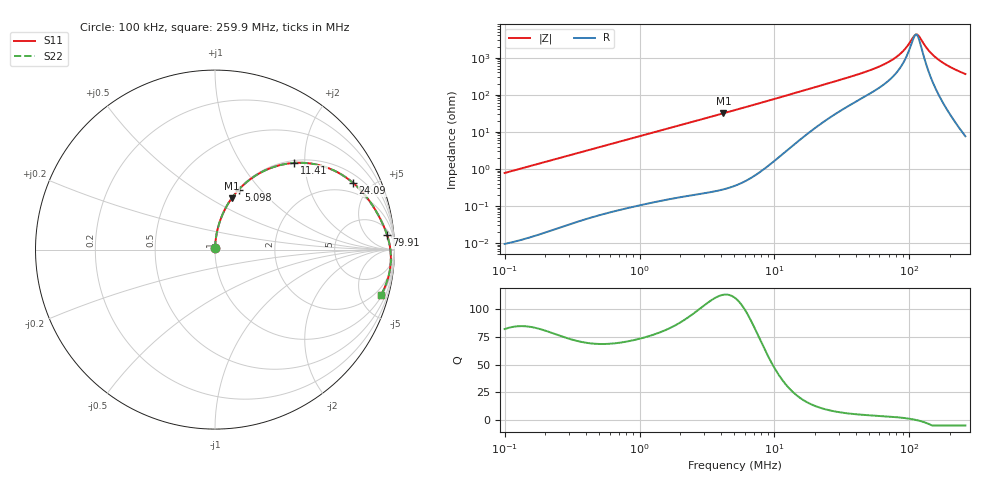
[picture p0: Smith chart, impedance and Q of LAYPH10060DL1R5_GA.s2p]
! LAYPH10060DL1R5_GA  S-PARAMETER MODEL  ( General Type )
! Model Generated by TAIYO YUDEN Corporation (http://www.ty-top.com)
! Version 3.0
! TAIYO YUDEN Control No. 180828NI43SB-FBB
! Copyright(c) 2017 TAIYO YUDEN CO.,LTD. All Rights Reserved.
! Product Description (link to TY-COMPAS)
! https://ds.yuden.co.jp/TYCOMPAS/or/detail?pn=LAYPH10060DL1R5NGA&u=M
! Products Name : Inductors
! Characteristics :
!  Inductance : 1.5 uH , SRF(min) : -Hz , DC Resistance(max) : 0.007 Ohm
!  Rated Current : Saturation :9 A , Temp Rise : 5.6 A (25 degC)
!  Case Size : 10.1 x 10.0 / 0.398 x 0.394 [mm/inch] , Thickness : 6 / 0.236 [mm/inch]
!  (Conditions: Temperature = 25 degC , DC Bias Current/Voltage = 0A / 0V)
! External Node Assignments :
!  1  o---GGG---o  2
! GND o---------o GND
! Frequency Range : 0.1MHz  -  259.929867MHz  [ 402 STEP ]
# MHz S RI R 50
! Freq[MHz].  S11 Real  S11 Imag  S21 Real  S21 Imag  S12 Real  S12 Imag  S22 Real  S22 Imag
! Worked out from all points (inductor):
!   401 points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, 100 kHz to 259.9 MHz, reference 50 ohm
!   read as one part in series: L = 1.23 uH near 104 kHz
!   highest Q = 113 at 4.188 MHz (marker M1), where L = 1.2 uH
!   self-resonance near 111.6 MHz
!   S11 on the Smith chart (normalised r, x): 100 kHz: 1.00, +0.02; 5.098 MHz: 1.01, +0.77; 11.41 MHz: 1.05, +1.77; 24.09 MHz: 1.41, +3.88; 79.91 MHz: 9, +19; 259.9 MHz: 1.15, -7.25
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0.1  0.000153 0.00771  0.9998 -0.00771  0.9998 -0.00771  0.000153 0.00771
0.37324  0.00122 0.0285  0.9988 -0.0285  0.9988 -0.0285  0.00122 0.0285
1.393082  0.0122 0.1038  0.9878 -0.1038  0.9878 -0.1038  0.0122 0.1038
2.463508  0.035 0.1786  0.965 -0.1786  0.965 -0.1786  0.035 0.1786
4.188482  0.0927 0.2856  0.9073 -0.2856  0.9073 -0.2856  0.0927 0.2856
5.098332  0.1314 0.3334  0.8686 -0.3334  0.8686 -0.3334  0.1314 0.3334
7.553894  0.2519 0.4276  0.7481 -0.4276  0.7481 -0.4276  0.2519 0.4276
11.41434  0.441 0.4829  0.559 -0.4829  0.559 -0.4829  0.441 0.4829
19.02902  0.6854 0.4294  0.3146 -0.4294  0.3146 -0.4294  0.6854 0.4294
24.09141  0.769 0.3719  0.231 -0.3719  0.231 -0.3719  0.769 0.3719
47.93603  0.9063 0.1987  0.0937 -0.1987  0.0937 -0.1987  0.9063 0.1987
59.50735  0.9314 0.1497  0.0686 -0.1497  0.0686 -0.1497  0.9314 0.1497
71.02397  0.9486 0.1097  0.0514 -0.1097  0.0514 -0.1097  0.9486 0.1097
79.9149  0.9583 0.0825  0.0417 -0.0825  0.0417 -0.0825  0.9583 0.0825
91.70389  0.9678 0.0496  0.0322 -0.0496  0.0322 -0.0496  0.9678 0.0496
107.321  0.9755 0.0102  0.0245 -0.0102  0.0245 -0.0102  0.9755 0.0102
113.8404  0.9775 -0.00512  0.0225 0.00512  0.0225 0.00512  0.9775 -0.00512
118.4051  0.9785 -0.0155  0.0215 0.0155  0.0215 0.0155  0.9785 -0.0155
138.5695  0.9797 -0.0587  0.0203 0.0587  0.0203 0.0587  0.9797 -0.0587
159.0112  0.9765 -0.0985  0.0235 0.0985  0.0235 0.0985  0.9765 -0.0985
197.395  0.9625 -0.1646  0.0375 0.1646  0.0375 0.1646  0.9625 -0.1646
259.9299  0.9247 -0.2537  0.0753 0.2537  0.0753 0.2537  0.9247 -0.2537
